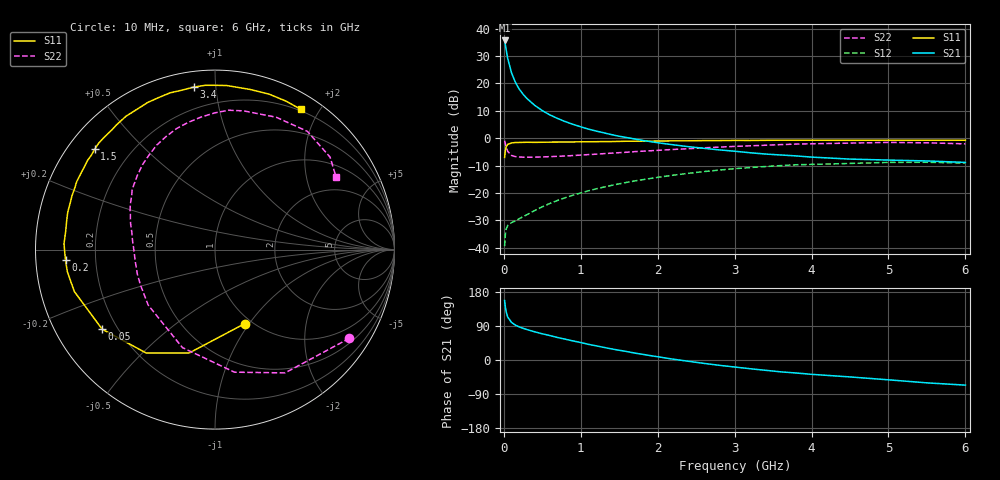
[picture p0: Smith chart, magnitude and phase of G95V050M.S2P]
! SIEMENS Small Signal Semiconductors
! BFG235
! Si NPN RF Bipolar Junction Transistor in SOT223
! VCE = 5 V  IC = 50 mA
! Common Emitter S-Parameters:  July  1994
# GHz  S  MA  R  50
!  f  S11  S21  S12  S22
! GHz  MAG  ANG  MAG  ANG  MAG  ANG  MAG  ANG
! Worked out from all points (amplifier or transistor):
!   40 points, 10 MHz to 6 GHz, reference 50 ohm
!   highest |S21| = 35.6 dB at 10 MHz (marker M1)
!   |S21| within 3 dB of that: start of sweep to 28.14 MHz
!   unconditionally stable (mu >= 1): 507.1 MHz to 1.291 GHz
!   at 200 MHz: K = 0.67, MSG = 23.6 dB, |S12| = -29.4 dB
!   at 1.5 GHz: K = 0.97, MSG = 8.7 dB, |S12| = -16.7 dB
!   at 6 GHz: K = 0.92, MSG = 0.1 dB, |S12| = -9.1 dB
!   S11 on the Smith chart (normalised r, x): 10 MHz: 0.93, -0.95; 50 MHz: 0.14, -0.31; 200 MHz: 0.09, -0.04; 1.5 GHz: 0.08, +0.36; 3.4 GHz: 0.08, +0.87; 6 GHz: 0.18, +1.77
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0.01  0.4445 -68.2  60.57 157.0  0.0107 69.4  0.8974 -33.4
0.02  0.5935 -104.0  50.38 139.5  0.0176 54.0  0.79 -60.4
0.03  0.6921 -123.7  41.33 127.4  0.0218 44.4  0.6914 -81.0
0.05  0.7693 -144.8  28.63 113.4  0.0255 34.4  0.5753 -108.4
0.1  0.8178 -163.4  15.49 99.1  0.0288 30.3  0.4839 -140.3
0.15  0.8319 -171.5  10.46 92.0  0.031 34.2  0.4598 -154.4
0.2  0.8349 -175.9  7.855 87.4  0.0339 37.5  0.4537 -162.4
0.25  0.8379 -179.5  6.33 83.6  0.0369 40.9  0.4495 -167.6
0.3  0.8418 177.7  5.287 80.4  0.0401 44.1  0.4492 -171.7
0.4  0.8382 173.0  3.98 74.4  0.0477 48.4  0.45 -177.3
0.5  0.842 168.9  3.178 69.1  0.0559 50.9  0.4543 178.4
0.6  0.8466 165.7  2.648 64.5  0.0645 52.3  0.4603 174.7
0.7  0.8475 162.1  2.281 59.3  0.0732 53.2  0.4668 171.4
0.9  0.8532 156.5  1.784 50.3  0.0911 52.4  0.4815 165.8
1.1  0.8598 150.0  1.461 41.3  0.1095 50.6  0.5012 160.2
1.5  0.873 140.2  1.083 25.7  0.1469 44.7  0.5435 149.5
2.2  0.8933 123.7  0.757 2.2  0.2107 30.6  0.6224 130.4
3.2  0.9072 101.8  0.542 -23.0  0.2907 7.0  0.7241 102.0
3.4  0.9131 97.5  0.513 -27.1  0.3034 2.0  0.7425 96.0
4.5  0.9134 77.6  0.415 -44.7  0.3459 -24.1  0.8125 65.2
5.5  0.9169 64.5  0.384 -60.3  0.3632 -46.5  0.8226 38.8
6  0.9164 58.6  0.361 -66.3  0.3519 -54.9  0.7869 31.1
